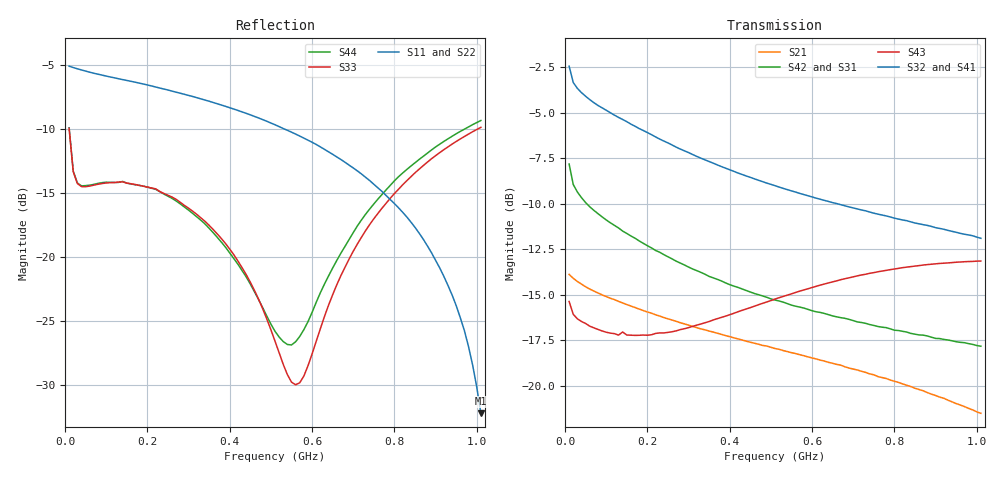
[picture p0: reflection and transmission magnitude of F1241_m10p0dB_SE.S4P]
! Integrated Device Technology
! Corporate Headquarters
! 6024 Silver Creek Valley Road
! San Jose, CA 95138  USA
! Phone:  1-408-284-8200
! Toll Free:  1-800-223-1366
! Webpage:  http://www.idt.com/
! Timing and RF Division
! 515 Groton Road, Suite 102
! Westford, MA 01886-6024
! Device:  F1241
! Description: Dual Intermediate Frequency Digital Variable Gain Amplifier
! Frequency:  10.0 -  500.00 MHz
! Package:  5x5 mm QFN Plastic Package: 32 pin
! Ports:  8 RF, 20 DC
!  Pin  1  = GA3  Pin 17  = RF OUT_B+
!  Pin  2  = GA4  Pin 18  = RF OUT_B-
!  Pin  3  = GA5  Pin 19  = STBY_B
!  Pin  4  = ISET_A  Pin 20  = Ground
!  Pin  5  = ISET_B  Pin 21  = Ground
!  Pin  6  = GB5  Pin 22  = STB_A
!  Pin  7  = GB4  Pin 23  = RF OUT_A-  = Port 4
!  Pin  8  = GB3  Pin 24  = RF OUT_A+  = Port 3
!  Pin  9  = GB2  Pin 25  = NO CONNECT
!  Pin 10  = GB1  Pin 26  = NO CONNECT
!  Pin 11  = RF IN_B+  Pin 27  = VCC
!  Pin 12  = RF IN_B-  Pin 28  = Ground
!  Pin 13  = Ground  Pin 29  = RF IN_A-  = Port 2
!  Pin 14  = VCC  Pin 30  = RF IN_A+  = Port 1
!  Pin 15  = NO CONNECT  Pin 31  = GA1
!  Pin 16  = NO CONNECT  Pin 32  = GA2
! State:  30
! Gain State:  -10.0 dB
! Voltages:  Vcc = +5.00 Volts  Icc approximately 160.0 mA or 80 mA per channel.
! Data:  The device was measured on a custom evaluation board which has
!  individual transmission lines to the RF pins.  Data was collected
!  using a calibrated network analyzer.  The evaluation board was
!  de-embedded using a port reference technique.
!  The reference plane is the edge of the package pin.
!  Only Channel A was measured.
!  This data is in single-ended operation.  If your needs are balanced
!  or differential S-parameters then this file needs to be used a
!  linear simulator.
! Misc:  Lot Code  160028MY
!  Action Tracker AT004
! Date Measured:  2014-08-14
! Date:  2014-08-28  MJV
! Note:
!  Integrated Device Technology supplies this data as a sample of measured
!  data at the package pin for this product.  Your particular data for this
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# Hz S dB R 50
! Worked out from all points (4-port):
!   101 points, 10 MHz to 1.01 GHz, reference 50 ohm
!   strongest paths, dB at 10 MHz, 260 MHz, 510 MHz, 760 MHz, 1.01 GHz:
!     S32: -2.4, -6.8, -9.0, -10.6, -11.9
!     S41: -2.4, -6.8, -9.1, -10.8, -12.2
!     S43: -15.4, -17.0, -15.2, -13.7, -13.1
!     S42: -7.8, -13.0, -15.3, -16.7, -17.8
!     S31: -7.8, -13.1, -15.4, -16.8, -17.9
!     S21: -13.9, -16.4, -18.0, -19.5, -21.5
!   lowest |S11| = -32.2 dB at 1.01 GHz (marker M1), VSWR 1.05, Z = 52.4 - j0.733 ohm
!   |S11| at or under -10 dB: 532.6 MHz to end of sweep
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1e7  -5.10 -3.8  -13.86 -7.8  -33.21 -2.9  -27.38 4.5
     -13.88 -7.8  -5.09 -3.7  -27.40 4.2  -33.24 -2.6
     -7.83 157.0  -2.44 164.6  -9.96 -45.7  -15.40 176.6
     -2.40 164.6  -7.81 157.2  -15.37 176.6  -9.91 -45.5
4e7  -5.40 -5.2  -14.40 -9.7  -34.01 -9.0  -27.79 -5.8
     -14.41 -9.6  -5.40 -5.1  -27.79 -5.4  -33.98 -9.3
     -9.68 156.5  -3.89 163.9  -14.50 -13.6  -16.52 166.9
     -3.85 163.8  -9.66 156.4  -16.47 166.8  -14.44 -13.3
3.8e8  -8.13 -16.6  -17.16 -33.2  -37.14 -11.1  -29.78 -17.9
       -17.17 -33.3  -8.11 -15.5  -29.60 -17.8  -37.12 -13.6
       -14.34 84.6  -7.96 120.6  -18.56 -8.3  -16.32 107.5
       -8.02 119.3  -14.24 83.7  -16.24 107.2  -18.84 -3.2
5.6e8  -10.40 -20.6  -18.21 -42.0  -36.93 -7.0  -29.88 -21.6
       -18.23 -42.2  -10.36 -19.2  -29.46 -22.5  -37.03 -9.9
       -15.72 57.3  -9.36 104.7  -29.96 56.7  -14.98 82.6
       -9.50 103.1  -15.63 55.7  -14.87 82.4  -26.61 68.1
7.1e8  -13.27 -23.8  -19.09 -49.5  -36.28 -6.1  -29.84 -26.4
       -19.13 -49.7  -13.30 -22.6  -29.19 -27.6  -36.43 -10.0
       -16.58 37.9  -10.28 92.4  -18.98 123.4  -14.10 63.4
       -10.49 90.8  -16.49 35.4  -13.96 63.3  -17.57 117.2
8.8e8  -19.12 -26.3  -20.30 -58.0  -35.38 -8.3  -29.83 -32.5
       -20.37 -58.2  -19.18 -26.6  -28.96 -35.0  -35.54 -11.2
       -17.34 18.8  -11.19 78.7  -12.59 124.3  -13.49 43.7
       -11.48 77.6  -17.26 15.3  -13.34 43.6  -11.89 120.4
1.01e9  -32.19 -16.5  -21.47 -64.4  -34.59 -11.6  -29.86 -37.5
        -21.51 -64.4  -32.54 -21.6  -28.85 -40.7  -34.73 -14.7
        -17.85 6.1  -11.90 68.7  -9.87 121.6  -13.29 30.2
        -12.18 67.8  -17.82 2.0  -13.15 30.2  -9.34 118.0
